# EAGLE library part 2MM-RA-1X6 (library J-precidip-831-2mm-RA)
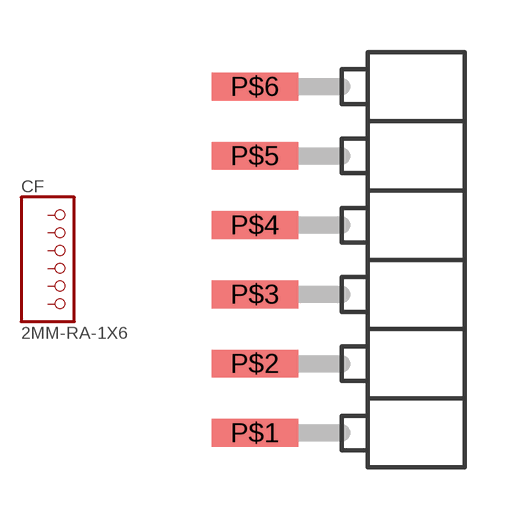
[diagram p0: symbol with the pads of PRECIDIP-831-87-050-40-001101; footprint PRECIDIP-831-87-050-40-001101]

Designator prefix CF

## 2MM-RA-1X6  [PRECIDIP-831-87-050-40-001101]
P$1  1  pas
P$2  2  pas
P$3  3  pas
P$4  4  pas
P$5  5  pas
P$6  6  pas

## Footprint PRECIDIP-831-87-050-40-001101 (pad centres in mm)
smd 2.5 x 0.8: P$1 -3.25,-5; P$2 -3.25,-3; P$3 -3.25,-1; P$4 -3.25,1; P$5 -3.25,3; P$6 -3.25,5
